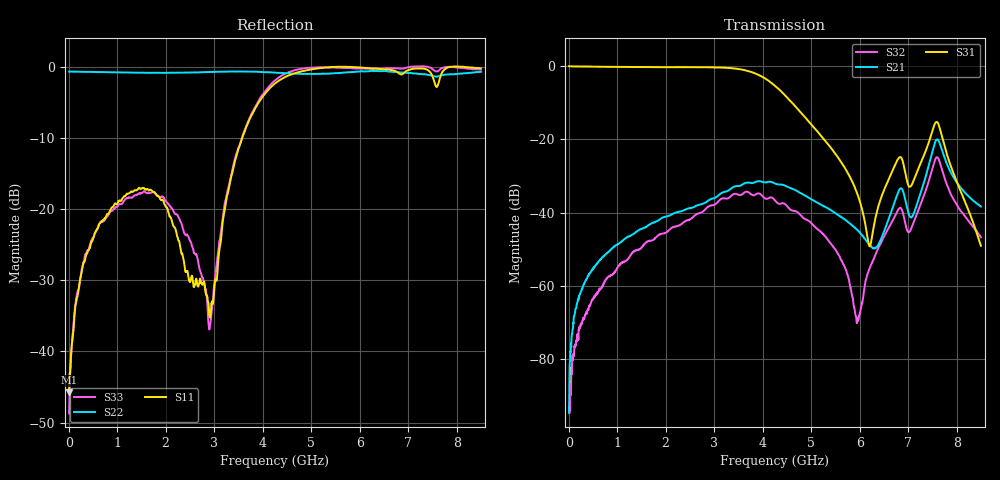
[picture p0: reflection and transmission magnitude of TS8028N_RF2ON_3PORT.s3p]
!Created with skrf (http://scikit-rf.org).
# GHz S RI R 50.0
!freq ReS11 ImS11 ReS12 ImS12 ReS13 ImS13
! ReS21 ImS21 ReS22 ImS22 ReS23 ImS23
! ReS31 ImS31 ReS32 ImS32 ReS33 ImS33
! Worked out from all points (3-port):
!   1601 points, 10 MHz to 8.5 GHz, reference 50 ohm
!   strongest paths, dB at 10 MHz, 2.132 GHz, 4.255 GHz, 6.378 GHz, 8.5 GHz:
!     S31: -0.1, -0.3, -5.4, -38.7, -49.0
!     S21: -94.5, -40.4, -32.0, -49.0, -38.3
!     S32: -91.8, -44.1, -36.6, -49.9, -46.7
!   lowest |S11| = -45.7 dB at 10 MHz (marker M1), VSWR 1.01, Z = 50.5 + j0.253 ohm
!   |S11| at or under -10 dB: start of sweep to 3.579 GHz
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0.01  0.00453 0.00251  -1.07e-05 4.21e-05  0.9928 -0.0127
      5.77e-06 1.79e-05  -0.922 0.00488  -1.44e-05 4.38e-06
      0.9928 -0.0129  4.7e-06 -2.52e-05  0.00214 0.00299
0.64675  -0.0438 -0.0665  -7.2e-05 0.00226  0.8638 -0.4522
         -6.1e-05 0.00227  -0.8974 0.1837  -0.000816 -0.000299
         0.8639 -0.4524  -0.000848 -0.000277  -0.019 -0.0777
2.222706  -0.0589 0.0338  0.00317 0.00959  -0.1407 -0.9523
          0.00317 0.0096  -0.7245 0.5451  -0.0027 0.00597
          -0.1407 -0.9522  -0.00264 0.00598  -0.0768 -0.0503
2.912519  0.00722 0.016  0.00704 0.0133  -0.6954 -0.6594
          0.0071 0.0133  -0.5798 0.709  0.00128 0.0123
          -0.6953 -0.6591  0.00127 0.0124  -0.0138 0.006
4.255  0.5449 0.5326  0.0248 -0.00366  -0.1942 0.5005
       0.0247 -0.00363  -0.3533 0.8364  0.0134 -0.00591
       -0.1947 0.4993  0.0135 -0.00596  0.7898 -0.1223
5.475437  0.9195 -0.3801  0.0062 -0.00797  0.0377 0.055
          0.00617 -0.00797  0.0578 0.8968  0.000602 -0.00326
          0.0378 0.0549  0.00057 -0.00326  0.5246 -0.8352
5.947694  0.8091 -0.5678  0.00405 -0.00422  0.0116 0.0143
          0.00404 -0.00423  0.1537 0.9098  0.0003 -0.000108
          0.0117 0.0144  0.000341 -0.000105  0.3792 -0.8913
6.213006  0.7374 -0.637  0.00337 -0.00126  -0.00224 0.00268
          0.00338 -0.00129  0.1862 0.9108  0.000677 0.00166
          -0.00225 0.0027  0.000691 0.00164  0.2954 -0.9198
7.582019  0.403 -0.5973  0.0981 -0.0115  -0.0728 0.1569
          0.0978 -0.0119  0.4712 0.7084  0.0526 -0.0203
          -0.0724 0.1566  0.0528 -0.0202  0.1162 -0.917
8.5  0.4468 -0.8638  -0.00145 -0.0121  0.00269 0.00229
     -0.00147 -0.0121  0.6867 0.6108  -0.00273 -0.00376
     0.00276 0.00222  -0.00275 -0.00373  0.0395 -0.9509
